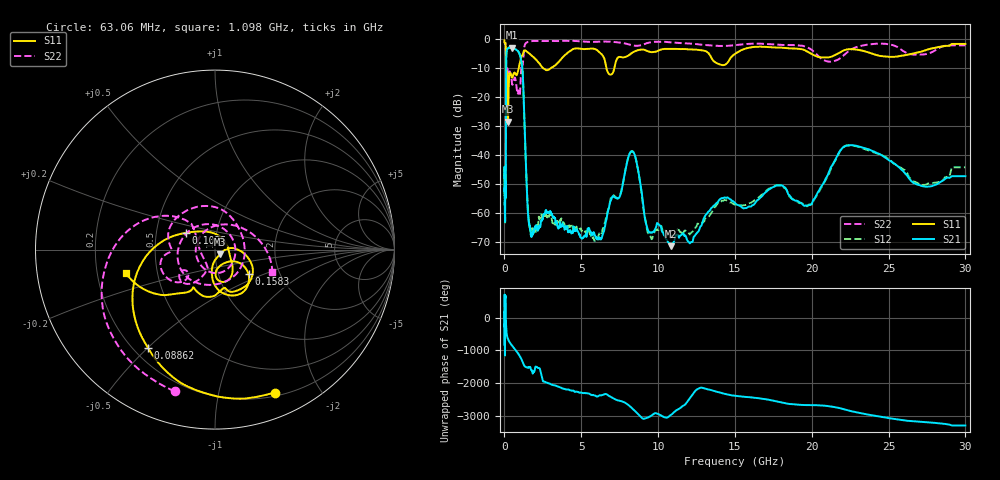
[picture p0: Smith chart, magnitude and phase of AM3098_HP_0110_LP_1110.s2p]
! Date/Time: Thu, Feb 28, 2019 8:38 AM
! Network Analyzer: Agilent Technologies E8364B Rev: A.07.50.67
! Sweep from 0.010 to 30.000 GHz, 1601 Points, Sweep Type: LOG
! Power Supply: 5.022 V, 0.002 A
# Hz S DB R 50
!freq MagS11 AngS11 MagS21 AngS21 MagS12 AngS12 MagS22 AngS22
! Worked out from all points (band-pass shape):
!   1601 points, 10 MHz to 30 GHz, reference 50 ohm
!   highest |S21| = -2.79 dB at 490.6 MHz (marker M1); lowest = -71.3 dB at 10.81 GHz (marker M2)
!   |S21| within 3 dB of the highest: 118.6 MHz to 1.028 GHz (909.9 MHz wide, 159 % of centre)
!   lowest |S11| = -28.3 dB at 237.5 MHz (marker M3), VSWR 1.08, Z = 52.9 - j2.69 ohm
!   |S11| at or under -10 dB: 99.93 MHz to 922.4 MHz (822.5 MHz wide, 161 % of centre); 2.535 GHz to 2.992 GHz (456.3 MHz wide, 16.5 % of centre); 6.641 GHz to 7.148 GHz (506.9 MHz wide, 7.35 % of centre)
!   |S22| runs from -22.1 to -0.5 dB; largest |S21 - S12| = 0.01
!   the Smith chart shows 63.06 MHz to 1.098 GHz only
!   S11 on the Smith chart (normalised r, x): 63.06 MHz: 0.24, -1.48; 88.62 MHz: 0.26, -0.50; 102.5 MHz: 0.71, +0.14; 158.3 MHz: 1.39, -0.40; 1.098 GHz: 0.33, -0.12
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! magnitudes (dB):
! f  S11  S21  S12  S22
! 10 MHz  -0.4  -47.6  -44.6  -0.6
! 38.04 MHz  -0.5  -57.4  -57.6  -1.0
! 63.06 MHz  -1.3  -52.2  -49.8  -1.7
! 88.62 MHz  -3.6  -43.6  -43.1  -3.9
! 102.5 MHz  -14.6  -14.7  -14.7  -19.3
! 144.7 MHz  -18.8  -3.9  -3.8  -14.0
! 158.3 MHz  -12.7  -3.6  -3.6  -11.7
! 237.5 MHz  -28.3  -3.0  -2.9  -12.0
! 311.2 MHz  -12.7  -2.9  -2.8  -11.3
! 490.6 MHz  -13.1  -2.8  -2.8  -15.3
! 550.5 MHz  -12.5  -3.0  -2.9  -15.2
! 1.098 GHz  -5.8  -7.6  -7.6  -9.3
! 1.567 GHz  -4.6  -62.3  -61.1  -0.8
! 2.084 GHz  -7.1  -65.2  -65.6  -0.5
! 6.171 GHz  -4.4  -68.2  -66.9  -0.7
! 7.926 GHz  -5.9  -43.8  -43.6  -1.5
! 8.459 GHz  -4.2  -39.5  -39.5  -2.2
! 9.49 GHz  -4.3  -66.6  -67.6  -1.0
! 10.81 GHz  -3.3  -71.3  -68.3  -1.0
! 19.7 GHz  -4.2  -57.3  -57.5  -2.7
! 22.67 GHz  -3.4  -36.5  -36.6  -3.2
! 30 GHz  -1.6  -47.2  -44.1  -2.0
